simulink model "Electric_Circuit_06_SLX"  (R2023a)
settings: Solver=ode23s  StartTime=0.0  StopTime=10.0  MaxStep=0.001  RelTol=1e-3
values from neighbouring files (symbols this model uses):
  C_4 = 0.001*F    (= 0.001)    [Electric_Circuit_06_EQN.m]    (also in Electric_Circuit_06_SLX_m.m; Electric_Circuit_01_EQN.m; Electric_Circuit_01_SLX_m.m; Electric_Circuit_09_EQN.m)
  C_6 = 0.001*F    (= 0.001)    [Electric_Circuit_06_EQN.m]    (also in Electric_Circuit_06_SLX_m.m; Electric_Circuit_01_EQN.m; Electric_Circuit_01_SLX_m.m; Electric_Circuit_03_EQN.m)
  I_2_0 = 0*A    (= 0)    [Electric_Circuit_06_SLX_m.m]    (also in Electric_Circuit_02_SLX_m.m; Electric_Circuit_03_SLX_m.m; Electric_Circuit_08_SLX_m.m; Electric_Circuit_09_SLX_m.m)
  I_5_0 = 0*A    (= 0)    [Electric_Circuit_06_SLX_m.m]    (also in BIG_EC_Simscape_SLX_m.m; Electric_Circuit_01_SLX_m.m; Electric_Circuit_09_SLX_m.m; Electric_Circuit_10_SLX_m.m)
  I_8_0 = 0*A    (= 0)    [Electric_Circuit_06_SLX_m.m]    (also in Electric_Circuit_02_SLX_m.m; Electric_Circuit_05_SLX_m.m; Electric_Circuit_07_SLX_m.m; Electric_Circuit_08_SLX_m.m)
  L_2 = 0.002*H    (= 0.002)    [Electric_Circuit_06_EQN.m]    (also in Electric_Circuit_06_SLX_m.m; Electric_Circuit_02_EQN.m; Electric_Circuit_02_SLX_m.m; Electric_Circuit_03_EQN.m)
  L_5 = 0.002*H    (= 0.002)    [Electric_Circuit_06_EQN.m]    (also in Electric_Circuit_06_SLX_m.m; BIG_EC_Simscape_EQN.m; BIG_EC_Simscape_SLX_m.m; Electric_Circuit_01_EQN.m)
  R_3 = 100*Ohm    (= 100)    [Electric_Circuit_06_EQN.m]    (also in Electric_Circuit_06_SLX_m.m; Electric_Circuit_01_EQN.m; Electric_Circuit_01_SLX_m.m; Electric_Circuit_02_EQN.m)
  R_7 = 100*Ohm    (= 100)    [Electric_Circuit_06_EQN.m]    (also in Electric_Circuit_06_SLX_m.m; BIG_EC_Simscape_EQN.m; BIG_EC_Simscape_SLX_m.m; Electric_Circuit_03_EQN.m)
  Ts = Tfin/Nr_Ts_Points    (= 0.0015708)    [Electric_Circuit_06_SLX_m.m]    (also in BIG_EC_Simscape_SLX_m.m = 0.0003; Car_Dumper_SLX_m.m = 0.0022779; Electric_Circuit_01_SLX_m.m = 0.005; Electric_Circuit_02_SLX_m.m = 0.000480145)
  V_1_0 = 10*V    (= 10)    [Electric_Circuit_06_SLX_m.m]    (also in BIG_EC_Simscape_SLX_m.m; Electric_Circuit_02_SLX_m.m; Electric_Circuit_03_SLX_m.m; Electric_Circuit_04_SLX_m.m)
  V_4_0 = 0*V    (= 0)    [Electric_Circuit_06_SLX_m.m]    (also in Electric_Circuit_01_SLX_m.m; Electric_Circuit_09_SLX_m.m)
  V_6_0 = 0*V    (= 0)    [Electric_Circuit_06_SLX_m.m]    (also in Electric_Circuit_01_SLX_m.m; Electric_Circuit_03_SLX_m.m; Electric_Circuit_08_SLX_m.m; Electric_Circuit_10_SLX_m.m)

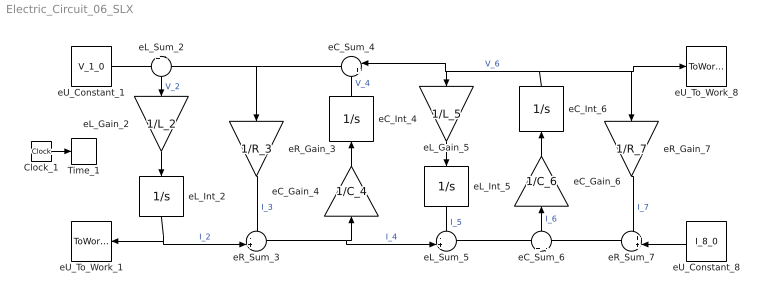
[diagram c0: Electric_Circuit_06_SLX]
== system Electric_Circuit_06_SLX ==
  Clock_1 : Clock
  Time_1 : ToWorkspace  VariableName=t  SaveFormat=Timeseries  SampleTime=Ts
  eC_Gain_4 : Gain  Gain=1/C_4  Multiplication=Matrix(K*u)
  eC_Gain_6 : Gain  Gain=1/C_6  Multiplication=Matrix(K*u)
  eC_Int_4 : Integrator  InitialCondition=V_4_0
  eC_Int_6 : Integrator  InitialCondition=V_6_0
  eC_Sum_4 : Sum  Inputs=|++
  eC_Sum_6 : Sum  Inputs=+|-
  eL_Gain_2 : Gain  Gain=1/L_2  Multiplication=Matrix(K*u)
  eL_Gain_5 : Gain  Gain=1/L_5  Multiplication=Matrix(K*u)
  eL_Int_2 : Integrator  InitialCondition=I_2_0
  eL_Int_5 : Integrator  InitialCondition=I_5_0
  eL_Sum_2 : Sum  Inputs=+|-
  eL_Sum_5 : Sum  Inputs=-+|
  eR_Gain_3 : Gain  Gain=1/R_3  Multiplication=Matrix(K*u)
  eR_Gain_7 : Gain  Gain=1/R_7  Multiplication=Matrix(K*u)
  eR_Sum_3 : Sum  Inputs=-+|
  eR_Sum_7 : Sum  Inputs=++|
  eU_Constant_1 : Constant  Value=V_1_0
  eU_Constant_8 : Constant  Value=I_8_0
  eU_To_Work_1 : ToWorkspace  VariableName=I_1_0  SaveFormat=Timeseries  SampleTime=Ts
  eU_To_Work_8 : ToWorkspace  VariableName=V_8_0  SaveFormat=Timeseries  SampleTime=Ts
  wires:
  eU_Constant_1/1 -> eL_Sum_2/1
  eC_Sum_4/1 -> eL_Sum_2/2, eR_Gain_3/1
  eL_Int_2/1 -> eU_To_Work_1/1, eR_Sum_3/2  "I_2"
  eL_Sum_2/1 -> eL_Gain_2/1  "V_2"
  eL_Gain_2/1 -> eL_Int_2/1
  eR_Sum_3/1 -> eC_Gain_4/1, eL_Sum_5/2  "I_4"
  eR_Gain_3/1 -> eR_Sum_3/1  "I_3"
  eC_Int_6/1 -> eC_Sum_4/1, eL_Gain_5/1, eU_To_Work_8/1, eR_Gain_7/1  "V_6"
  eC_Gain_4/1 -> eC_Int_4/1
  eC_Int_4/1 -> eC_Sum_4/2  "V_4"
  eL_Sum_5/1 -> eC_Sum_6/1
  eL_Gain_5/1 -> eL_Int_5/1
  eL_Int_5/1 -> eL_Sum_5/1  "I_5"
  eR_Sum_7/1 -> eC_Sum_6/2
  eC_Sum_6/1 -> eC_Gain_6/1  "I_6"
  eC_Gain_6/1 -> eC_Int_6/1
  eU_Constant_8/1 -> eR_Sum_7/2
  eR_Gain_7/1 -> eR_Sum_7/1  "I_7"
  Clock_1/1 -> Time_1/1
